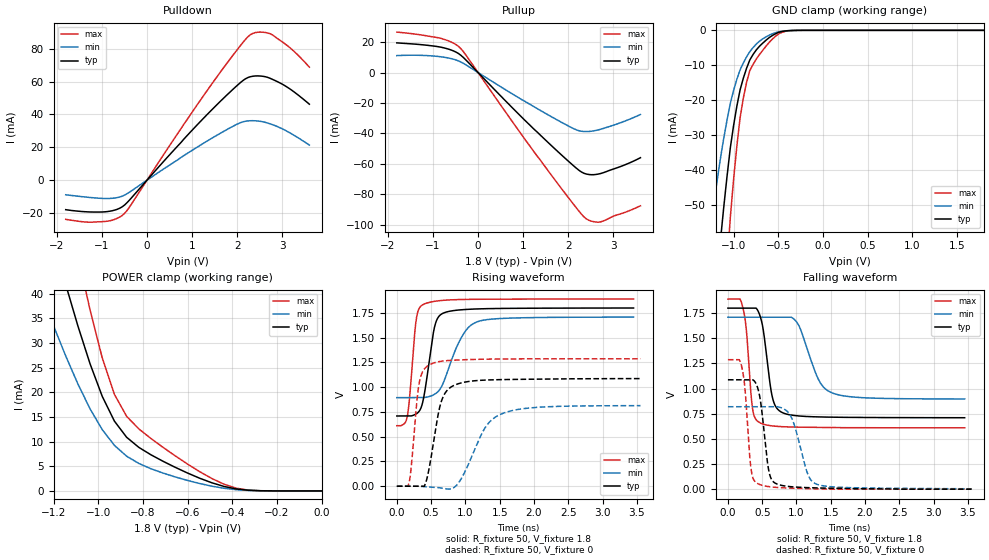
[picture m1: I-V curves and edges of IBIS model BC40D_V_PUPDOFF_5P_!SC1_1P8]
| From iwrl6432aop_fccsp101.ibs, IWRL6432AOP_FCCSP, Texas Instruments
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|   Model Cell BC40D_V_PUPDOFF_5P_!SC1_1P8
|BC40D_V_PUPDOFF_5P_!SC1_1P8
[Model]   BC40D_V_PUPDOFF_5P_!SC1_1P8
Model_type   I/O
Polarity   Non-Inverting
Enable   Active-Low
Vinl =  0.63
Vinh =  1.17
Cref =  15pF
Rref =  100.0000M
Vref =  0V
Vmeas =  0.9
C_comp   2.233931p   2.204415p   2.290246p
|[Input load] weak_pupdoff
|[Output drive] fast
|[supplytol] 5
|[temp] ind
[Model Spec]
Vinl   0.63   0.5985   0.6615
Vinh   1.17   1.1115   1.2285
[Temperature Range]   25   125   -40
[Voltage Range]   1.8   1.71   1.89
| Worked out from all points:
|   slope of the pulldown table from 0 to 0.27 V, typ, clamps not added: 32.2 ohm
|   slope of the pullup table from 0 to 0.27 V, typ, clamps not added: 32.5 ohm
|   GND clamp passes 1 mA (typ) near -0.53 V on its own axis
|   POWER clamp passes 1 mA (typ) near -0.44 V on its own axis
|   rising waveform, R_fixture 50, V_fixture 1.8: 20-80 % time 141ps typ, 294ps min, 91.6ps max; typ from 0.709 V to 1.8 V
|   rising waveform, R_fixture 50, V_fixture 0: 20-80 % time 174ps typ, 350ps min, 104ps max; typ from 0 V to 1.09 V
|   falling waveform, R_fixture 50, V_fixture 1.8: 20-80 % time 128ps typ, 263ps min, 86.3ps max; typ from 1.8 V to 0.71 V
|   falling waveform, R_fixture 50, V_fixture 0: 20-80 % time 111ps typ, 196ps min, 82.8ps max; typ from 1.09 V to 0 V
| Nom Voltages:
|   VDD=1.1, VDDS=1.8, VDDS18=1.8, ESD_BIASFET=0, VSS=0, VSSS=0
| Min Voltages:
|   VDD=1.045, VDDS=1.71, VDDS18=1.71, ESD_BIASFET=0, VSS=0, VSSS=0
| Max Voltages:
|   VDD=1.16, VDDS=1.89, VDDS18=1.89, ESD_BIASFET=0, VSS=0, VSSS=0
[POWER_clamp]
|   voltage   I(typ)   I(min)   I(max)
-1.8V     158.8mA    112.5mA    219.7mA
-1.255V   59.93mA    39.99mA    84.86mA
-1.127V   39.08mA    25.5mA     55.75mA
-1.055V   28.36mA    18.34mA    40.41mA
-981.8mV  19.18mA    12.43mA    26.98mA
-927.3mV  14.16mA    9.239mA    19.58mA
-872.7mV  10.89mA    7.049mA    15.14mA
-818.2mV  8.843mA    5.579mA    12.59mA
-600mV    3.63mA     2.128mA    5.45mA
-436.4mV  903.9uA    539uA      1.358mA
-327.3mV  138.2uA    94.87uA    160.3uA
0V        19.3nA     133.7nA    230.3nA
[Pulldown]
|   voltage   I(typ)   I(min)   I(max)
-1.8V     -17.92mA   -8.85mA    -23.8mA
-1.309V   -19.26mA   -10.37mA   -25.5mA
-927.3mV  -19.22mA   -11.12mA   -25.08mA
-654.5mV  -17.65mA   -10.56mA   -23.13mA
-490.9mV  -14.97mA   -8.985mA   -20.05mA
1.364V    40.78mA    24.32mA    55.7mA
2.073V    59.41mA    35mA       81.91mA
2.291V    62.96mA    36.2mA     88.48mA
2.509V    63.41mA    35.84mA    90.12mA
2.782V    61.38mA    33.82mA    88.42mA
3.218V    54.59mA    28.02mA    79.45mA
3.6V      46.26mA    21.39mA    68.79mA
[Pullup]
|   voltage   I(typ)   I(min)   I(max)
-1.8V     19.47mA    11.11mA    26.55mA
-818.2mV  16.61mA    10.32mA    22.37mA
-545.5mV  14.21mA    8.765mA    19.31mA
-381.8mV  11.35mA    6.928mA    15.71mA
1.255V    -37.58mA   -22.7mA    -52.59mA
2.127V    -61.49mA   -36.97mA   -86.91mA
2.291V    -65.3mA    -38.55mA   -92.97mA
2.4V      -66.65mA   -38.77mA   -96.07mA
2.564V    -67.08mA   -38.3mA    -97.93mA
2.727V    -66.24mA   -37.15mA   -97.99mA
3.273V    -60.4mA    -31.68mA   -91.65mA
3.6V      -55.92mA   -27.55mA   -87.52mA
[GND_clamp]
|   voltage   I(typ)   I(min)   I(max)
-1.8V     -270.2mA   -170.2mA   -430.1mA
-1.255V   -91.66mA   -55.91mA   -148.4mA
-1.145V   -59.91mA   -36.45mA   -97.09mA
-1.109V   -50.48mA   -30.83mA   -81.55mA
-1.073V   -41.73mA   -25.65mA   -67.05mA
-1.036V   -33.66mA   -20.92mA   -53.59mA
-927.3mV  -17.07mA   -11.35mA   -25.04mA
-854.5mV  -10.86mA   -7.617mA   -14.91mA
-781.8mV  -6.919mA   -4.945mA   -9.771mA
-636.4mV  -2.823mA   -1.868mA   -4.529mA
-381.8mV  -84.73uA   -78.82uA   -126.1uA
1.8V      19.3nA     350.9nA    215.8nA
[Ramp]
| variable   typ   min   max
dV/dt_f 0.66582249/0.13069096n 0.49991745/0.26945059n 0.77756876/87.983914p
dV/dt_r 0.66457062/0.17691361n 0.50985211/0.36481894n   0.781455/0.10527652n
R_load = 50
[Rising Waveform]
R_fixture = 50
V_fixture = 1.8
V_fixture_min = 1.71
V_fixture_max = 1.89
|   time   V(typ)   V(min)   V(max)
0s        709.3mV    894.4mV    611.2mV
149.8ps   709.3mV    894.4mV    694.5mV
187.6ps   709.3mV    894.4mV    904mV
280.8ps   729.4mV    894.4mV    1.671V
386.4ps   875.3mV    895.7mV    1.836V
549.1ps   1.604V     928.2mV    1.867V
678.4ps   1.748V     1.045V     1.877V
932.6ps   1.781V     1.491V     1.885V
1.179ns   1.791V     1.662V     1.888V
3.453ns   1.8V       1.708V     1.89V
[Rising Waveform]
R_fixture = 50
V_fixture = 0
V_fixture_min = 0
V_fixture_max = 0
|   time   V(typ)   V(min)   V(max)
0s        0V         0V         0V
177.5ps   0V         0V         32.05mV
322.8ps   0V         0V         1.027V
401.4ps   0V         -4.654mV   1.183V
480.7ps   214.8mV    -8.338mV   1.228V
647.3ps   852.1mV    -17.62mV   1.262V
851ps     1.023V     -3.712mV   1.273V
1.28ns    1.072V     582.8mV    1.283V
1.512ns   1.077V     725.9mV    1.285V
3.554ns   1.087V     813.8mV    1.287V
[Falling Waveform]
R_fixture = 50
V_fixture = 1.8
V_fixture_min = 1.71
V_fixture_max = 1.89
|   time   V(typ)   V(min)   V(max)
0s        1.8V       1.71V      1.89V
215.1ps   1.8V       1.71V      1.814V
269.6ps   1.8V       1.71V      1.578V
357.6ps   1.8V       1.71V      808.4mV
465ps     1.73V      1.71V      660.9mV
646.5ps   919.6mV    1.71V      629mV
789ps     762.9mV    1.71V      621.3mV
1.018ns   728.9mV    1.647V     616.7mV
1.502ns   715.8mV    962.5mV    612.4mV
3.453ns   710.3mV    896.7mV    610mV
[Falling Waveform]
R_fixture = 50
V_fixture = 0
V_fixture_min = 0
V_fixture_max = 0
|   time   V(typ)   V(min)   V(max)
0s        1.088V     819.6mV    1.287V
199.2ps   1.088V     819.6mV    1.224V
249.5ps   1.088V     819.6mV    994mV
335.9ps   1.088V     819.6mV    208.3mV
436ps     1.003V     819.6mV    54.75mV
592.2ps   198.2mV    819.6mV    25.53mV
703.6ps   54.91mV    819.6mV    17.69mV
926.3ps   23.91mV    713.1mV    10.12mV
1.286ns   12.59mV    51.37mV    3.156mV
3.554ns   0V         3.787mV    0V
